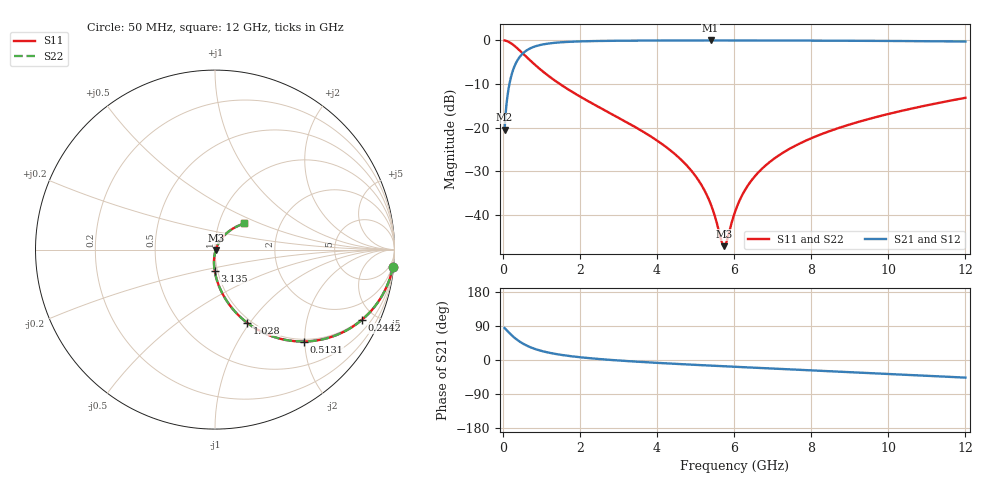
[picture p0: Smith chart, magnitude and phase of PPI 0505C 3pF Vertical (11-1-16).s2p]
# GHz S MA R 50
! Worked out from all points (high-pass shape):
!   1601 points, 50 MHz to 12 GHz, reference 50 ohm
!   highest |S21| = -0.04 dB at 5.39 GHz (marker M1); lowest = -20.5 dB at 50 MHz (marker M2)
!   |S21| within 3 dB of the highest: 519.4 MHz to end of sweep
!   lowest |S11| = -47.2 dB at 5.741 GHz (marker M3), VSWR 1.01, Z = 50.4 - j0.136 ohm
!   |S11| at or under -10 dB: 1.48 GHz to end of sweep
!   |S22| runs from -47.2 to 0.0 dB; largest |S21 - S12| = 0
!   S11 on the Smith chart (normalised r, x): 50 MHz: 1, -20; 244.2 MHz: 0.95, -4.19; 513.1 MHz: 0.95, -1.98; 1.028 GHz: 0.95, -0.97; 3.135 GHz: 0.97, -0.24; 12 GHz: 1.32, +0.40
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0.05  0.9955 -5.6  0.09466 84.4  0.09466 84.4  0.9955 -5.6
0.1545625  0.9593 -16.8  0.2821 73.1  0.2821 73.1  0.9593 -16.8
0.2441875  0.9065 -25.6  0.4216 64.3  0.4216 64.3  0.9065 -25.6
0.5130625  0.7127 -45.9  0.7003 44.0  0.7003 44.0  0.7127 -45.9
0.7520625  0.5664 -57.5  0.8225 32.3  0.8225 32.3  0.5664 -57.5
1.028406  0.4441 -66.4  0.894 23.4  0.894 23.4  0.4441 -66.4
2.044156  0.2216 -82.4  0.9723 6.9  0.9723 6.9  0.2216 -82.4
3.134594  0.1206 -90.6  0.9892 -2.2  0.9892 -2.2  0.1206 -90.6
4.038312  0.06924 -94.7  0.9937 -7.7  0.9937 -7.7  0.06924 -94.7
4.874812  0.03276 -95.2  0.9951 -12.2  0.9951 -12.2  0.03276 -95.2
5.166094  0.02156 -92.6  0.9953 -13.7  0.9953 -13.7  0.02156 -92.6
5.390156  0.01345 -86.5  0.9953 -14.8  0.9953 -14.8  0.01345 -86.5
5.673969  0.005007 -46.0  0.9953 -16.2  0.9953 -16.2  0.005007 -46.0
5.741187  0.004373 -17.9  0.9953 -16.5  0.9953 -16.5  0.004373 -17.9
5.815875  0.005077 13.0  0.9952 -16.9  0.9952 -16.9  0.005077 13.0
6.025  0.01078 47.5  0.9951 -17.9  0.9951 -17.9  0.01078 47.5
6.316281  0.02027 57.5  0.9948 -19.3  0.9948 -19.3  0.02027 57.5
6.719594  0.03355 60.6  0.9942 -21.2  0.9942 -21.2  0.03355 60.6
7.27975  0.05184 60.6  0.9932 -23.8  0.9932 -23.8  0.05184 60.6
8.019156  0.07592 58.7  0.9913 -27.3  0.9913 -27.3  0.07592 58.7
10.01331  0.1435 50.8  0.9827 -36.7  0.9827 -36.7  0.1435 50.8
12  0.2192 41.6  0.9676 -46.5  0.9676 -46.5  0.2192 41.6
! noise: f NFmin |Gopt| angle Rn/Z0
0.05  0.0007536  0.9371  1.617  0.002671
1.372  0.005726  0.7618  4.767  0.004867
2.701  0.009184  0.7153  8.345  0.006338
4.031  0.01226  0.6876  11.95  0.007547
5.36  0.01517  0.6692  15.53  0.00866
6.682  0.01801  0.6568  19.04  0.009749
8.012  0.02088  0.6488  22.51  0.01088
9.341  0.02383  0.6445  25.92  0.01208
10.67  0.0269  0.6433  29.27  0.0134
12  0.03015  0.6449  32.55  0.01488
